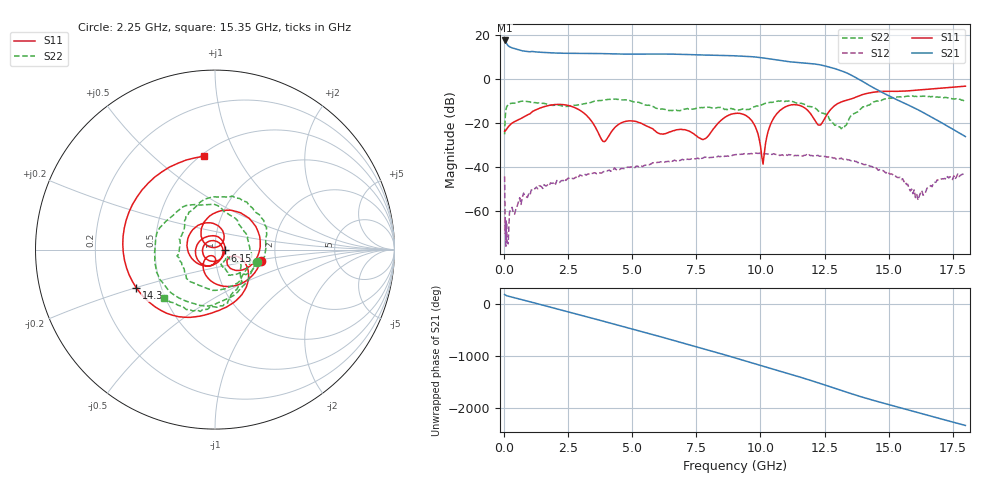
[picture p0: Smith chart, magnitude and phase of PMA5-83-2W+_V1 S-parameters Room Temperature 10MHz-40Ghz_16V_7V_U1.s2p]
!Mini-Circuits Laboratory
!S-Parameters
!Model: US-AMP-1
!Run / Lot / Date Code: N/A /  / N/A
!Fixture: ON TB-
!Network Analyzer: NFA N8975A;  Serial number: 74408
!Date: 12/1/2023 at 8:06:11 AM
!No.: Unit# 2 (#4)
!Tested with:
!Condition 5: Vdd = +16V; Vg2= +7V; Idd= 400mA
# Hz  S  dB  R  50
!Frequency  S11 dB  S11 Deg  S21 dB  S21 Deg  S12 dB  S12 Deg  S22 dB  S22 Deg
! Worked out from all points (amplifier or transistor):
!   368 points, 10 MHz to 18 GHz, reference 50 ohm
!   highest |S21| = 17.5 dB at 20 MHz (marker M1)
!   |S21| within 3 dB of that: start of sweep to 226.6 MHz
!   unconditionally stable (mu >= 1): start of sweep to end of sweep
!   at 2.7 GHz: K = 21.55, MAG = 12.2 dB, |S12| = -45.4 dB
!   at 8.85 GHz: K = 7.82, MAG = 10.9 dB, |S12| = -35.1 dB
!   at 18 GHz: K = 732.23, MAG = -23.0 dB, |S12| = -43.6 dB
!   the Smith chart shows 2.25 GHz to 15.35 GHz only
!   S11 on the Smith chart (normalised r, x): 2.25 GHz: 1.66, -0.23; 6.15 GHz: 1.12, -0.01; 14.3 GHz: 0.36, -0.20; 15.35 GHz: 0.52, +0.75
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1e7  -23.75 -2.1  17.37 177.1  -44.33 118.7  -25.20 -59.3
2e7  -23.79 -3.0  17.52 173.9  -54.89 -73.0  -21.17 -89.4
5e8  -18.82 -146.0  13.48 101.1  -57.85 42.4  -10.66 141.2
1.15e9  -14.46 113.8  12.41 19.8  -49.90 -43.1  -10.74 67.8
2.25e9  -11.62 -14.5  11.72 -121.5  -46.17 -179.1  -12.26 -16.6
3.05e9  -15.01 -96.6  11.65 134.6  -44.06 81.7  -11.42 -62.1
4e9  -27.36 -92.2  11.49 9.0  -41.92 -36.3  -9.37 -131.9
4.75e9  -19.23 -134.3  11.32 -89.7  -40.53 -136.6  -9.47 165.4
5.4e9  -20.48 145.5  11.34 -175.8  -39.82 144.0  -11.28 113.0
6.05e9  -24.82 18.6  11.37 96.3  -37.90 62.4  -13.62 63.9
6.15e9  -25.01 -4.9  11.35 82.7  -37.75 49.9  -13.64 56.7
7.35e9  -24.68 131.4  11.04 -82.0  -36.36 -106.3  -13.70 -32.8
8.1e9  -23.72 -66.0  10.81 174.5  -35.67 154.3  -13.13 -102.9
9.05e9  -15.62 144.7  10.52 40.1  -34.36 27.3  -14.05 177.1
9.85e9  -23.23 46.5  9.93 -76.8  -33.78 -85.8  -12.24 131.8
1.05e10  -18.11 128.7  8.88 -172.1  -34.01 -174.4  -10.52 81.4
1.12e10  -11.76 42.4  7.76 87.5  -34.50 88.3  -10.11 22.9
1.205e10  -17.36 -50.6  6.91 -39.8  -35.01 -34.6  -12.87 -35.7
1.43e10  -6.23 -154.2  -3.26 -32.7  -39.68 -23.3  -11.38 -71.0
1.505e10  -5.59 129.9  -7.86 -134.4  -43.26 -110.0  -8.63 -115.7
1.535e10  -5.61 96.6  -9.58 -174.4  -44.80 -138.1  -8.14 -136.8
1.8e10  -3.27 159.5  -26.19 -167.7  -43.59 49.2  -9.88 45.7
